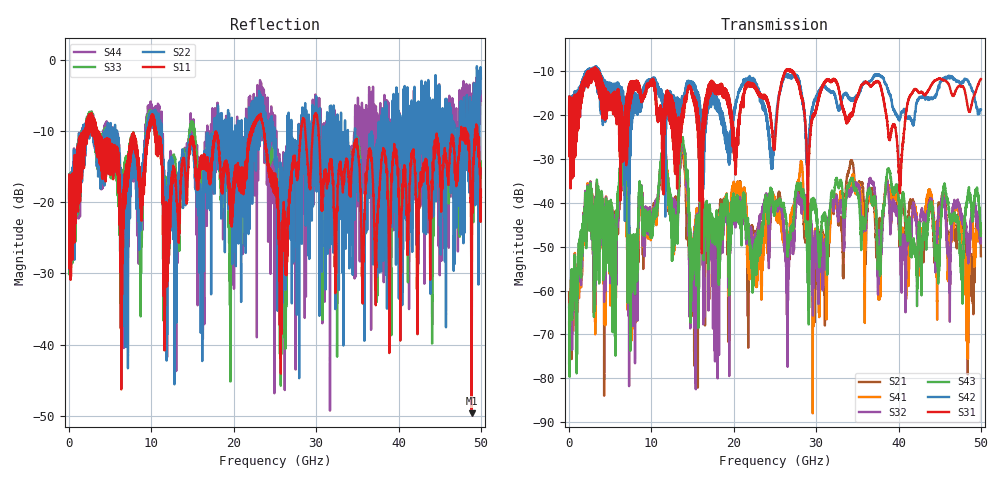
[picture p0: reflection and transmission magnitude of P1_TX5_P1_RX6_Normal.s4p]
!Keysight Technologies,N5225B,MY57041031,A.13.20.10
!Date: Friday, May 31, 2019 11:22:39
!Correction: S11(Full 4 Port(1,2,3,4))
!S12(Full 4 Port(1,2,3,4))
!S13(Full 4 Port(1,2,3,4))
!S14(Full 4 Port(1,2,3,4))
!S21(Full 4 Port(1,2,3,4))
!S22(Full 4 Port(1,2,3,4))
!S23(Full 4 Port(1,2,3,4))
!S24(Full 4 Port(1,2,3,4))
!S31(Full 4 Port(1,2,3,4))
!S32(Full 4 Port(1,2,3,4))
!S33(Full 4 Port(1,2,3,4))
!S34(Full 4 Port(1,2,3,4))
!S41(Full 4 Port(1,2,3,4))
!S42(Full 4 Port(1,2,3,4))
!S43(Full 4 Port(1,2,3,4))
!S44(Full 4 Port(1,2,3,4))
!S4P File: Measurements: <S11,S12,S13,S14>,
!<S21,S22,S23,S24>,
!<S31,S32,S33,S34>,
!<S41,S42,S43,S44>:
# Hz S  dB  R 50.0
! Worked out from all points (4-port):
!   5000 points, 10 MHz to 50 GHz, reference 50 ohm
!   strongest paths, dB at 10 MHz, 12.51 GHz, 25.01 GHz, 37.51 GHz, 50 GHz:
!     S31: -19.4, -23.0, -26.1, -12.3, -11.7
!     S42: -19.3, -15.6, -23.3, -10.8, -18.8
!     S43: -63.9, -42.4, -40.3, -54.5, -46.3
!     S32: -76.6, -41.0, -40.3, -60.9, -49.0
!     S41: -67.2, -42.7, -40.8, -54.9, -46.9
!     S21: -60.4, -41.9, -39.5, -46.9, -52.1
!   lowest |S11| = -49.6 dB at 48.87 GHz (marker M1), VSWR 1.01, Z = 50.3 - j0.14 ohm
!   |S11| at or under -10 dB: 3.502 GHz to 9.556 GHz (6.054 GHz wide, 92.7 % of centre); 10.5 GHz to 22.11 GHz (11.6 GHz wide, 71.2 % of centre); 30.29 GHz to 47.6 GHz (17.3 GHz wide, 44.4 % of centre)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
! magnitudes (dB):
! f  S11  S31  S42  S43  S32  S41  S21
! 10 MHz  -19.8  -19.4  -19.3  -63.9  -76.6  -67.2  -60.4
! 2.15 GHz  -9.9  -12.4  -12.4  -39.0  -38.2  -38.4  -37.8
! 11.51 GHz  -32.9  -23.5  -21.1  -26.5  -26.6  -26.5  -26.9
! 17.92 GHz  -10.6  -15.3  -17.7  -41.7  -50.6  -52.3  -50.1
! 34.29 GHz  -15.8  -19.8  -16.5  -34.5  -36.8  -34.6  -30.4
! 48.87 GHz  -49.6  -17.6  -13.8  -41.8  -41.9  -45.5  -55.7
! 50 GHz  -18.3  -11.7  -18.8  -46.3  -49.0  -46.9  -52.1
